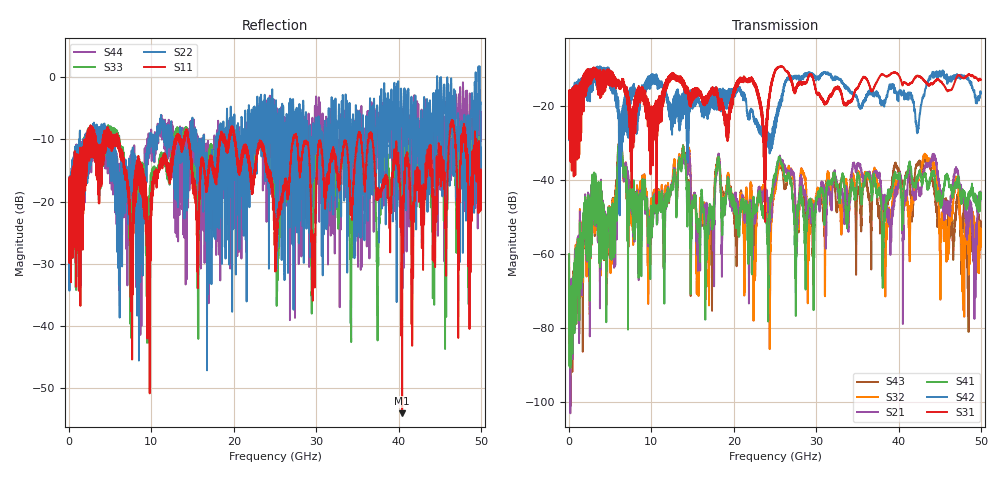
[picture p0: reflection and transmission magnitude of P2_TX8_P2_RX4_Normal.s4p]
!Keysight Technologies,N5225B,MY57041031,A.13.20.10
!Date: Friday, May 31, 2019 11:33:10
!Correction: S11(Full 4 Port(1,2,3,4))
!S12(Full 4 Port(1,2,3,4))
!S13(Full 4 Port(1,2,3,4))
!S14(Full 4 Port(1,2,3,4))
!S21(Full 4 Port(1,2,3,4))
!S22(Full 4 Port(1,2,3,4))
!S23(Full 4 Port(1,2,3,4))
!S24(Full 4 Port(1,2,3,4))
!S31(Full 4 Port(1,2,3,4))
!S32(Full 4 Port(1,2,3,4))
!S33(Full 4 Port(1,2,3,4))
!S34(Full 4 Port(1,2,3,4))
!S41(Full 4 Port(1,2,3,4))
!S42(Full 4 Port(1,2,3,4))
!S43(Full 4 Port(1,2,3,4))
!S44(Full 4 Port(1,2,3,4))
!S4P File: Measurements: <S11,S12,S13,S14>,
!<S21,S22,S23,S24>,
!<S31,S32,S33,S34>,
!<S41,S42,S43,S44>:
# Hz S  dB  R 50.0
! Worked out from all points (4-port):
!   5000 points, 10 MHz to 50 GHz, reference 50 ohm
!   strongest paths, dB at 10 MHz, 12.51 GHz, 25.01 GHz, 37.51 GHz, 50 GHz:
!     S31: -19.3, -11.7, -10.3, -12.8, -12.8
!     S42: -19.6, -27.7, -24.2, -16.9, -16.6
!     S41: -60.1, -41.6, -38.6, -44.0, -44.3
!     S21: -67.5, -41.3, -40.5, -39.1, -45.0
!     S32: -60.3, -41.2, -43.0, -41.9, -56.1
!     S43: -68.9, -41.3, -40.4, -47.4, -54.4
!   lowest |S11| = -54.0 dB at 40.44 GHz (marker M1), VSWR 1.00, Z = 50.2 + j0.0725 ohm
!   |S11| at or under -10 dB: 20.17 GHz to 27.19 GHz (7.016 GHz wide, 29.6 % of centre); 27.67 GHz to 35.04 GHz (7.367 GHz wide, 23.5 % of centre); 36.82 GHz to 46.17 GHz (9.35 GHz wide, 22.5 % of centre)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
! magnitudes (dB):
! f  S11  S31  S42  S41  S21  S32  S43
! 10 MHz  -19.6  -19.3  -19.6  -60.1  -67.5  -60.3  -68.9
! 6.21 GHz  -11.9  -15.3  -25.5  -28.3  -28.9  -28.4  -27.8
! 16.81 GHz  -16.6  -17.1  -21.7  -56.0  -48.2  -56.4  -57.0
! 18.1 GHz  -12.2  -17.7  -20.8  -34.3  -33.2  -33.3  -34.0
! 22.55 GHz  -15.6  -14.7  -23.6  -49.1  -51.8  -65.0  -57.9
! 40.44 GHz  -54.0  -14.2  -16.3  -53.6  -47.4  -44.9  -41.7
! 50 GHz  -14.9  -12.8  -16.6  -44.3  -45.0  -56.1  -54.4
